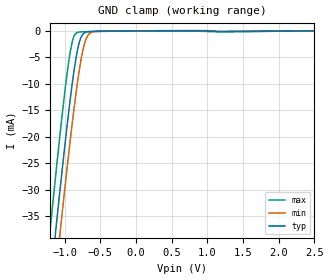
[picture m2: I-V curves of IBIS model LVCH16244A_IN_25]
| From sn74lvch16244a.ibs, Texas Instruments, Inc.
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[Model]   LVCH16244A_IN_25
Model_type  Input
Vinl=0.7
Vinh=1.7
| variable   typ   min   max
C_comp   3.12pF   2.47pF   4.24pF
[Temperature Range]   40   100   -40
| Ambient temperature   25   85   -40
[Voltage range]   2.5   2.3   2.7
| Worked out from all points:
|   GND clamp passes 1 mA (typ) near -0.76 V on its own axis
[GND Clamp]
| LVCH16244A_IN_25
|   Voltage   I(typ)   I(min)   I(max)
-5V       -584.7mA   -591.5mA   -576.3mA
-1.225V   -51.14mA   -59.35mA   -40.63mA
-1.2V     -47.82mA   -56.04mA   -37.29mA
-1.13V    -38.61mA   -46.84mA   -28.07mA
-1.07V    -30.89mA   -39.09mA   -20.41mA
-1.05V    -28.36mA   -36.54mA   -17.93mA
-955mV    -16.84mA   -24.77mA   -7.115mA
-885mV    -9.242mA   -16.64mA   -1.704mA
-775mV    -1.412mA   -5.909mA   -194.2uA
-710mV    -281.2uA   -1.988mA   -160.8uA
-645mV    -112.1uA   -448.6uA   -140.8uA
2.5V      7.214pA    38.7nA     -765.8pA
